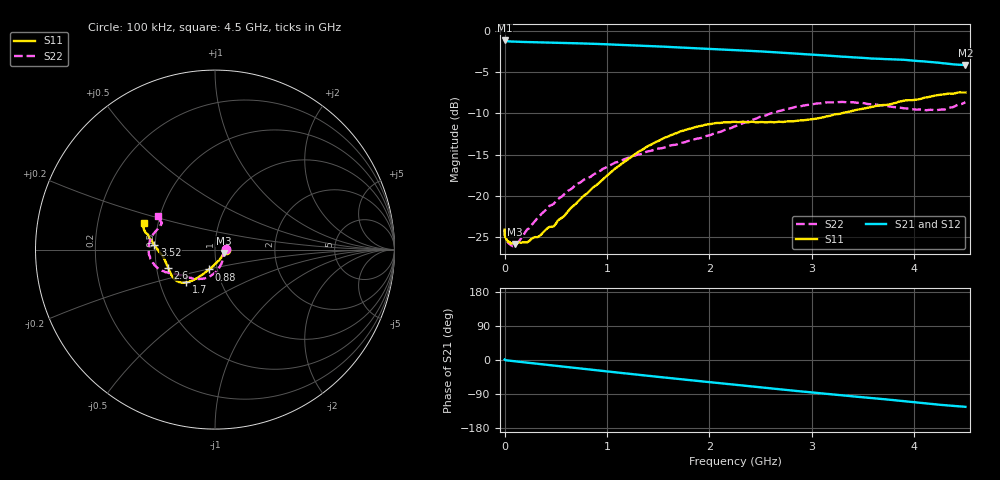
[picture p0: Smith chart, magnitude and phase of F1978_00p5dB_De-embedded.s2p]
! Integrated Device Technology
! Corporate Headquarters
! 6024 Silver Creek Valley Road
! San Jose, CA 95138  USA
! Phone:  1-408-284-8200
! Toll Free:  1-800-223-1366
! Webpage:  http://www.idt.com/
! Timing and RF Division
! 515 Groton Road, Suite 102
! Westford, MA 01886-6024
! Device:  F1978
! Description: 6-bit, 75 ohm, 0.5 dB Digital Step Attenuator
! Frequency:  5.0 MHz -  3.00 GHz
! Package:  4x4 mm QFN Plastic Package: 20 pin
! Ports:  2 RF, 11 DC
!  Pin  1  = D5 (16 dB)
!  Pin  2  = RF1  =  Port 1
!  Pin  3  = Serial Data In (DATA)
!  Pin  4  = Serial Clock (CLK)
!  Pin  5  = Serial Latch Enable (LE)
!  Pin  6  = VDD
!  Pin  7  = NC
!  Pin  8  = NC
!  Pin  9  = NC
!  Pin 10  = GND
!  Pin 11  = GND
!  Pin 12  = NC
!  Pin 13  = VMODE
!  Pin 14  = RF2  =  Port 2
!  Pin 15  = D4 (8 dB)
!  Pin 16  = D3 (4 dB)
!  Pin 17  = D2 (2 dB)
!  Pin 18  = NC
!  Pin 19  = D1 (1 dB)
!  Pin 20  = D0 (0.5 dB)
! State:  1
! Atten State:  0.5 dB
! Voltage:  +3.30 Volts
! Current:  0.568 mA
! Data:  The device was measured on a F1975 evaluation board which has
!  individual transmission lines to the RF pins.  Data was collected
!  using a calibrated network analyzer.  The evaluation board was
!  de-embedded using Automatic Fixture Removal (AFR).
!  The reference plane is the edge of the package pin.
! Misc:
!  Action Tracker AT0416
! Date Measured:  2018-02-08
! Date:  2018-03-26  MJV
! Note:
!  Integrated Device Technology supplies this data as a sample of measured
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# GHz S dB R 75
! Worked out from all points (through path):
!   291 points, 100 kHz to 4.5 GHz, reference 75 ohm
!   highest |S21| = -1.17 dB at 100 kHz (marker M1); lowest = -4.1 dB at 4.5 GHz (marker M2)
!   group delay of S21, straight-line fit = 77.4 ps
!   lowest |S11| = -25.8 dB at 100 MHz (marker M3), VSWR 1.11, Z = 82.5 - j3.01 ohm
!   |S11| at or under -10 dB: start of sweep to 3.29 GHz
!   |S22| runs from -26.1 to -8.6 dB; largest |S21 - S12| = 0.00026
!   S11 on the Smith chart (normalised r, x): 100 kHz: 1.13, +0.00; 880 MHz: 0.92, -0.20; 1.7 GHz: 0.68, -0.26; 2.6 GHz: 0.57, -0.12; 3.52 GHz: 0.49, +0.03; 4.5 GHz: 0.42, +0.15
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0.0001  -24.04 0.1  -1.17 1.2  -1.17 1.2  -24.01 0.8
0.0009  -24.58 -1.6  -1.21 1.0  -1.21 1.0  -24.60 -0.3
0.002  -24.76 -1.4  -1.23 0.8  -1.22 0.8  -24.74 -0.6
0.02  -25.30 -6.2  -1.26 -0.9  -1.26 -0.9  -25.42 -6.9
0.1  -25.78 -20.7  -1.32 -3.4  -1.32 -3.4  -25.99 -24.4
0.22  -25.59 -40.0  -1.36 -7.0  -1.36 -7.0  -24.04 -45.4
0.44  -23.72 -68.8  -1.43 -13.6  -1.43 -13.6  -21.16 -65.4
0.48  -23.64 -74.4  -1.45 -14.7  -1.45 -14.7  -20.94 -69.1
0.76  -20.11 -99.7  -1.54 -23.0  -1.54 -23.0  -18.16 -87.0
0.88  -18.80 -106.1  -1.58 -26.5  -1.58 -26.5  -17.30 -94.0
1.28  -14.87 -121.0  -1.77 -38.2  -1.77 -38.2  -15.06 -113.0
1.52  -13.22 -126.9  -1.90 -45.1  -1.90 -45.1  -14.22 -122.7
1.7  -12.27 -131.4  -2.02 -50.1  -2.02 -50.1  -13.65 -130.6
1.96  -11.37 -138.1  -2.17 -57.3  -2.17 -57.3  -12.76 -140.6
2.26  -11.03 -147.2  -2.34 -65.5  -2.33 -65.5  -11.51 -149.3
2.6  -11.04 -159.1  -2.57 -74.9  -2.57 -74.9  -9.99 -158.0
3.02  -10.68 -172.7  -2.90 -86.1  -2.90 -86.1  -8.87 -171.0
3.28  -10.03 -179.1  -3.12 -92.9  -3.11 -92.9  -8.61 179.2
3.52  -9.38 175.4  -3.30 -99.0  -3.30 -99.0  -8.79 171.2
3.76  -8.90 171.2  -3.44 -104.8  -3.44 -104.8  -9.16 163.9
4.22  -7.80 165.0  -3.84 -117.3  -3.83 -117.3  -9.61 153.4
4.5  -7.47 159.2  -4.14 -123.6  -4.14 -123.6  -8.65 149.7
